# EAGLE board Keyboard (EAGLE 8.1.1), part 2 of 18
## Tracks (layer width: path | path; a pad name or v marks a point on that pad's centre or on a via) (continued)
S$778
  Bottom 0: 246.88,2.82 246.83,2.94
S$779
  Bottom 0: 246.83,2.94 261.31,2.94
S$780
  Bottom 0: 261.31,2.94 261.38,2.95
S$781
  Bottom 0: 261.38,2.95 261.44,2.96
S$782
  Bottom 0: 261.44,2.96 261.51,2.99
S$783
  Bottom 0: 261.51,2.99 261.57,3.03
S$784
  Bottom 0: 261.57,3.03 261.62,3.07
S$785
  Bottom 0: 261.62,3.07 269.2,10.64
S$786
  Bottom 0: 269.2,10.64 269.29,10.6
S$787
  Bottom 0: 269.29,10.6 269.6,10.58
S$788
  Bottom 0: 269.6,10.58 269.89,10.65
S$789
  Bottom 0: 269.89,10.65 270.15,10.8
S$790
  Bottom 0: 270.15,10.8 270.36,11.02
S$791
  Bottom 0: 270.36,11.02 270.44,11.19
S$792
  Bottom 0: 270.44,11.19 270.47,11.14
S$793
  Bottom 0: 270.47,11.14 270.52,11.09
S$794
  Bottom 0: 270.52,11.09 276.91,4.69
S$795
  Bottom 0: 276.91,4.69 276.96,4.65
S$796
  Bottom 0: 276.96,4.65 277.02,4.61
S$797
  Bottom 0: 277.02,4.61 277.09,4.58
S$798
  Bottom 0: 277.09,4.58 277.15,4.56
S$799
  Bottom 0: 277.15,4.56 277.22,4.56
S$800
  Bottom 0: 277.22,4.56 280.74,4.56
S$801
  Bottom 0: 280.74,4.56 280.76,4.49
S$802
  Bottom 0: 280.76,4.49 280.93,4.18
S$803
  Bottom 0: 280.93,4.18 281.17,3.92
S$804
  Bottom 0: 281.17,3.92 281.46,3.74
S$805
  Bottom 0: 281.46,3.74 281.8,3.63
S$806
  Bottom 0: 281.8,3.63 282.15,3.61
S$807
  Bottom 0: 282.15,3.61 282.45,3.67
S$808
  Bottom 0: 282.45,3.67 282.56,3.63
S$809
  Bottom 0: 282.56,3.63 282.91,3.61
S$810
  Bottom 0: 282.91,3.61 283.25,3.67
S$811
  Bottom 0: 283.25,3.67 283.57,3.82
S$812
  Bottom 0: 283.57,3.82 283.84,4.05
S$813
  Bottom 0: 283.84,4.05 284.05,4.33
S$814
  Bottom 0: 284.05,4.33 284.17,4.66
S$815
  Bottom 0: 284.17,4.66 284.22,5
S$816
  Bottom 0: 284.22,5 284.17,5.35
S$817
  Bottom 0: 284.17,5.35 284.05,5.67
S$818
  Bottom 0: 284.05,5.67 283.84,5.96
S$819
  Bottom 0: 283.84,5.96 283.57,6.18
S$820
  Bottom 0: 283.57,6.18 283.25,6.33
S$821
  Bottom 0: 283.25,6.33 282.91,6.39
S$822
  Bottom 0: 282.91,6.39 282.56,6.37
S$823
  Bottom 0: 282.56,6.37 282.45,6.34
S$824
  Bottom 0: 282.45,6.34 282.15,6.39
S$825
  Bottom 0: 282.15,6.39 281.8,6.37
S$826
  Bottom 0: 281.8,6.37 281.46,6.27
S$827
  Bottom 0: 281.46,6.27 281.17,6.08
S$828
  Bottom 0: 281.17,6.08 280.93,5.82
S$829
  Bottom 0: 280.93,5.82 280.76,5.51
S$830
  Bottom 0: 280.76,5.51 280.74,5.44
S$831
  Bottom 0: 280.74,5.44 279.89,5.44
S$832
  Bottom 0: 279.89,5.44 280.27,5.65
S$833
  Bottom 0: 280.27,5.65 280.62,5.93
S$834
  Bottom 0: 280.62,5.93 280.9,6.28
S$835
  Bottom 0: 280.9,6.28 281.12,6.67
S$836
  Bottom 0: 281.12,6.67 281.24,7.1
S$837
  Bottom 0: 281.24,7.1 281.29,7.55
S$838
  Bottom 0: 281.29,7.55 281.24,7.99
S$839
  Bottom 0: 281.24,7.99 281.12,8.42
S$840
  Bottom 0: 281.12,8.42 280.9,8.82
S$841
  Bottom 0: 280.9,8.82 280.62,9.16
S$842
  Bottom 0: 280.62,9.16 280.27,9.45
S$843
  Bottom 0: 280.27,9.45 279.87,9.66
S$844
  Bottom 0: 279.87,9.66 279.62,9.74
S$845
  Bottom 0: 279.62,9.74 284.97,9.74
S$846
  Bottom 0: 284.97,9.74 289.73,4.98
S$847
  Bottom 0: 289.73,4.98 289.53,4.97
S$848
  Bottom 0: 289.53,4.97 289.25,4.85
S$849
  Bottom 0: 289.25,4.85 289.01,4.67
S$850
  Bottom 0: 289.01,4.67 288.85,4.42
S$851
  Bottom 0: 288.85,4.42 288.75,4.13
S$852
  Bottom 0: 288.75,4.13 288.75,3.82
S$853
  Bottom 0: 288.75,3.82 288.85,3.53
S$854
  Bottom 0: 288.85,3.53 289.01,3.28
S$855
  Bottom 0: 289.01,3.28 289.25,3.1
S$856
  Bottom 0: 289.25,3.1 289.53,2.98
S$857
  Bottom 0: 289.53,2.98 289.83,2.96
S$858
  Bottom 0: 289.83,2.96 290.13,3.03
S$859
  Bottom 0: 290.13,3.03 290.4,3.18
S$860
  Bottom 0: 290.4,3.18 290.6,3.4
S$861
  Bottom 0: 290.6,3.4 290.66,3.53
S$862
  Bottom 0: 290.66,3.53 293.86,3.53
S$863
  Bottom 0: 293.86,3.53 293.63,3.28
S$864
  Bottom 0: 293.63,3.28 293.45,2.97
S$865
  Bottom 0: 293.45,2.97 293.43,2.9
S$866
  Bottom 0: 293.43,2.9 289.08,2.9
S$867
  Bottom 0: 289.08,2.9 288.34,3.65
S$868
  Bottom 0: 288.34,3.65 288.35,3.67
S$869
  Bottom 0: 288.35,3.67 288.4,3.98
S$870
  Bottom 0: 288.4,3.98 288.35,4.28
S$871
  Bottom 0: 288.35,4.28 288.22,4.55
S$872
  Bottom 0: 288.22,4.55 288.02,4.77
S$873
  Bottom 0: 288.02,4.77 287.75,4.92
S$874
  Bottom 0: 287.75,4.92 287.46,4.99
S$875
  Bottom 0: 287.46,4.99 287.15,4.97
S$876
  Bottom 0: 287.15,4.97 286.88,4.85
S$877
  Bottom 0: 286.88,4.85 286.64,4.67
S$878
  Bottom 0: 286.64,4.67 286.47,4.42
S$879
  Bottom 0: 286.47,4.42 286.38,4.13
S$880
  Bottom 0: 286.38,4.13 286.38,3.82
S$881
  Bottom 0: 286.38,3.82 286.47,3.53
S$882
  Bottom 0: 286.47,3.53 286.64,3.28
S$883
  Bottom 0: 286.64,3.28 286.88,3.1
S$884
  Bottom 0: 286.88,3.1 287.15,2.98
S$885
  Bottom 0: 287.15,2.98 287.46,2.96
S$886
  Bottom 0: 287.46,2.96 287.71,3.02
S$887
  Bottom 0: 287.71,3.02 288.58,2.15
S$888
  Bottom 0: 288.58,2.15 288.63,2.11
S$889
  Bottom 0: 288.63,2.11 288.7,2.06
S$890
  Bottom 0: 288.7,2.06 288.76,2.04
S$891
  Bottom 0: 288.76,2.04 288.82,2.02
S$892
  Bottom 0: 288.82,2.02 288.9,2.02
S$893
  Bottom 0: 288.9,2.02 293.43,2.02
S$894
  Bottom 0: 293.43,2.02 293.45,1.95
S$895
  Bottom 0: 293.45,1.95 293.63,1.64
S$896
  Bottom 0: 293.63,1.64 293.87,1.38
S$897
  Bottom 0: 293.87,1.38 294.16,1.2
S$898
  Bottom 0: 294.16,1.2 294.49,1.09
S$899
  Bottom 0: 294.49,1.09 294.84,1.07
S$900
  Bottom 0: 294.84,1.07 295.14,1.12
S$901
  Bottom 0: 295.14,1.12 295.25,1.09
S$902
  Bottom 0: 295.25,1.09 295.6,1.07
S$903
  Bottom 0: 295.6,1.07 295.95,1.13
S$904
  Bottom 0: 295.95,1.13 296.26,1.28
S$905
  Bottom 0: 296.26,1.28 296.53,1.51
S$906
  Bottom 0: 296.53,1.51 296.74,1.79
S$907
  Bottom 0: 296.74,1.79 296.87,2.12
S$908
  Bottom 0: 296.87,2.12 296.91,2.46
S$909
  Bottom 0: 296.91,2.46 296.87,2.81
S$910
  Bottom 0: 296.87,2.81 296.74,3.13
S$911
  Bottom 0: 296.74,3.13 296.53,3.42
S$912
  Bottom 0: 296.53,3.42 296.39,3.53
S$913
  Bottom 0: 296.39,3.53 296.52,3.53
S$914
  Bottom 0: 296.52,3.53 296.55,3.49
S$915
  Bottom 0: 296.55,3.49 296.59,3.43
S$916
  Bottom 0: 296.59,3.43 297.44,2.58
S$917
  Bottom 0: 297.44,2.58 297.5,2.54
S$918
  Bottom 0: 297.5,2.54 297.56,2.5
S$919
  Bottom 0: 297.56,2.5 297.62,2.47
S$920
  Bottom 0: 297.62,2.47 297.69,2.46
S$921
  Bottom 0: 297.69,2.46 297.76,2.45
S$922
  Bottom 0: 297.76,2.45 298.36,2.45
S$923
  Bottom 0: 298.36,2.45 298.66,2.15
S$924
  Bottom 0: 298.66,2.15 298.72,2.11
S$925
  Bottom 0: 298.72,2.11 298.78,2.06
S$926
  Bottom 0: 298.78,2.06 298.84,2.04
S$927
  Bottom 0: 298.84,2.04 298.91,2.02
S$928
  Bottom 0: 298.91,2.02 298.98,2.02
S$929
  Bottom 0: 298.98,2.02 312.48,2.02
S$930
  Bottom 0: 312.48,2.02 312.5,1.95
S$931
  Bottom 0: 312.5,1.95 312.67,1.64
S$932
  Bottom 0: 312.67,1.64 312.91,1.38
S$933
  Bottom 0: 312.91,1.38 313.2,1.2
S$934
  Bottom 0: 313.2,1.2 313.54,1.09
S$935
  Bottom 0: 313.54,1.09 313.89,1.07
S$936
  Bottom 0: 313.89,1.07 314.19,1.12
S$937
  Bottom 0: 314.19,1.12 314.3,1.09
S$938
  Bottom 0: 314.3,1.09 314.65,1.07
S$939
  Bottom 0: 314.65,1.07 314.99,1.13
S$940
  Bottom 0: 314.99,1.13 315.31,1.28
S$941
  Bottom 0: 315.31,1.28 315.58,1.51
S$942
  Bottom 0: 315.58,1.51 315.79,1.79
S$943
  Bottom 0: 315.79,1.79 315.91,2.12
S$944
  Bottom 0: 315.91,2.12 315.96,2.46
S$945
  Bottom 0: 315.96,2.46 315.91,2.81
S$946
  Bottom 0: 315.91,2.81 315.79,3.13
S$947
  Bottom 0: 315.79,3.13 315.58,3.42
S$948
  Bottom 0: 315.58,3.42 315.31,3.64
S$949
  Bottom 0: 315.31,3.64 314.99,3.79
S$950
  Bottom 0: 314.99,3.79 314.65,3.85
S$951
  Bottom 0: 314.65,3.85 314.3,3.83
S$952
  Bottom 0: 314.3,3.83 314.19,3.8
S$953
  Bottom 0: 314.19,3.8 313.89,3.85
S$954
  Bottom 0: 313.89,3.85 313.54,3.83
S$955
  Bottom 0: 313.54,3.83 313.2,3.73
S$956
  Bottom 0: 313.2,3.73 312.91,3.54
S$957
  Bottom 0: 312.91,3.54 312.67,3.28
S$958
  Bottom 0: 312.67,3.28 312.5,2.97
S$959
  Bottom 0: 312.5,2.97 312.48,2.9
S$960
  Bottom 0: 312.48,2.9 299.17,2.9
S$961
  Bottom 0: 299.17,2.9 298.86,3.21
S$962
  Bottom 0: 298.86,3.21 298.81,3.25
S$963
  Bottom 0: 298.81,3.25 298.75,3.29
S$964
  Bottom 0: 298.75,3.29 298.69,3.31
S$965
  Bottom 0: 298.69,3.31 298.62,3.33
S$966
  Bottom 0: 298.62,3.33 298.55,3.33
S$967
  Bottom 0: 298.55,3.33 297.94,3.33
S$968
  Bottom 0: 297.94,3.33 297.35,3.93
S$969
  Bottom 0: 297.35,3.93 297.35,3.98
S$970
  Bottom 0: 297.35,3.98 297.32,4.11
S$971
  Bottom 0: 297.32,4.11 297.26,4.23
S$972
  Bottom 0: 297.26,4.23 297.16,4.33
S$973
  Bottom 0: 297.16,4.33 297.04,4.4
S$974
  Bottom 0: 297.04,4.4 296.9,4.42
S$975
  Bottom 0: 296.9,4.42 290.66,4.42
S$976
  Bottom 0: 290.66,4.42 290.6,4.55
S$977
  Bottom 0: 290.6,4.55 290.52,4.63
S$978
  Bottom 0: 290.52,4.63 299.77,4.63
S$979
  Bottom 0: 299.77,4.63 299.8,4.49
S$980
  Bottom 0: 299.8,4.49 299.98,4.18
S$981
  Bottom 0: 299.98,4.18 300.21,3.92
S$982
  Bottom 0: 300.21,3.92 300.51,3.74
S$983
  Bottom 0: 300.51,3.74 300.84,3.63
S$984
  Bottom 0: 300.84,3.63 301.19,3.61
S$985
  Bottom 0: 301.19,3.61 301.5,3.67
S$986
  Bottom 0: 301.5,3.67 301.6,3.63
S$987
  Bottom 0: 301.6,3.63 301.95,3.61
S$988
  Bottom 0: 301.95,3.61 302.3,3.67
S$989
  Bottom 0: 302.3,3.67 302.61,3.82
S$990
  Bottom 0: 302.61,3.82 302.88,4.05
S$991
  Bottom 0: 302.88,4.05 303.09,4.33
S$992
  Bottom 0: 303.09,4.33 303.22,4.66
S$993
  Bottom 0: 303.22,4.66 303.26,5
S$994
  Bottom 0: 303.26,5 303.22,5.35
S$995
  Bottom 0: 303.22,5.35 303.09,5.67
S$996
  Bottom 0: 303.09,5.67 302.88,5.96
S$997
  Bottom 0: 302.88,5.96 302.61,6.18
S$998
  Bottom 0: 302.61,6.18 302.3,6.33
S$999
  Bottom 0: 302.3,6.33 301.95,6.39
S$1000
  Bottom 0: 301.95,6.39 301.6,6.37
S$1001
  Bottom 0: 301.6,6.37 301.5,6.34
S$1002
  Bottom 0: 301.5,6.34 301.19,6.39
S$1003
  Bottom 0: 301.19,6.39 301.02,6.38
S$1004
  Bottom 0: 301.02,6.38 301.02,15.1
S$1005
  Bottom 0: 301.02,15.1 301.22,14.91
S$1006
  Bottom 0: 301.22,14.91 301.51,14.77
S$1007
  Bottom 0: 301.51,14.77 301.83,14.7
S$1008
  Bottom 0: 301.83,14.7 302.15,14.72
S$1009
  Bottom 0: 302.15,14.72 302.46,14.83
S$1010
  Bottom 0: 302.46,14.83 302.73,15.01
S$1011
  Bottom 0: 302.73,15.01 302.93,15.27
S$1012
  Bottom 0: 302.93,15.27 303.06,15.57
S$1013
  Bottom 0: 303.06,15.57 303.11,15.89
S$1014
  Bottom 0: 303.11,15.89 303.06,16.21
S$1015
  Bottom 0: 303.06,16.21 303.05,16.23
S$1016
  Bottom 0: 303.05,16.23 303.75,16.93
S$1017
  Bottom 0: 303.75,16.93 312.77,16.93
S$1018
  Bottom 0: 312.77,16.93 312.65,16.87
S$1019
  Bottom 0: 312.65,16.87 312.42,16.64
S$1020
  Bottom 0: 312.42,16.64 312.25,16.37
S$1021
  Bottom 0: 312.25,16.37 312.16,16.05
S$1022
  Bottom 0: 312.16,16.05 312.16,15.73
S$1023
  Bottom 0: 312.16,15.73 312.25,15.41
S$1024
  Bottom 0: 312.25,15.41 312.42,15.14
S$1025
  Bottom 0: 312.42,15.14 312.65,14.92
S$1026
  Bottom 0: 312.65,14.92 312.94,14.77
S$1027
  Bottom 0: 312.94,14.77 313.26,14.7
S$1028
  Bottom 0: 313.26,14.7 313.58,14.72
S$1029
  Bottom 0: 313.58,14.72 313.61,14.73
S$1030
  Bottom 0: 313.61,14.73 314.57,13.77
S$1031
  Bottom 0: 314.57,13.77 314.19,13.77
S$1032
  Bottom 0: 314.19,13.77 314.11,13.76
S$1033
  Bottom 0: 314.11,13.76 314.04,13.72
S$1034
  Bottom 0: 314.04,13.72 313.98,13.66
S$1035
  Bottom 0: 313.98,13.66 313.94,13.59
S$1036
  Bottom 0: 313.94,13.59 313.93,13.52
S$1037
  Bottom 0: 313.93,13.52 313.93,11.74
S$1038
  Bottom 0: 313.93,11.74 313.94,11.66
S$1039
  Bottom 0: 313.94,11.66 313.98,11.59
S$1040
  Bottom 0: 313.98,11.59 314.04,11.53
S$1041
  Bottom 0: 314.04,11.53 314.11,11.49
S$1042
  Bottom 0: 314.11,11.49 314.19,11.48
S$1043
  Bottom 0: 314.19,11.48 316.59,11.48
S$1044
  Bottom 0: 316.59,11.48 316.67,11.49
S$1045
  Bottom 0: 316.67,11.49 316.74,11.53
S$1046
  Bottom 0: 316.74,11.53 316.8,11.59
S$1047
  Bottom 0: 316.8,11.59 316.84,11.66
S$1048
  Bottom 0: 316.84,11.66 316.85,11.74
S$1049
  Bottom 0: 316.85,11.74 316.85,11.96
S$1050
  Bottom 0: 316.85,11.96 316.86,11.93
S$1051
  Bottom 0: 316.86,11.93 317.1,11.74
S$1052
  Bottom 0: 317.1,11.74 317.38,11.63
S$1053
  Bottom 0: 317.38,11.63 317.69,11.61
S$1054
  Bottom 0: 317.69,11.61 317.81,11.64
S$1055
  Bottom 0: 317.81,11.64 317.9,11.58
S$1056
  Bottom 0: 317.9,11.58 318.21,11.49
S$1057
  Bottom 0: 318.21,11.49 318.53,11.49
S$1058
  Bottom 0: 318.53,11.49 318.84,11.58
S$1059
  Bottom 0: 318.84,11.58 319.12,11.76
S$1060
  Bottom 0: 319.12,11.76 319.33,12
S$1061
  Bottom 0: 319.33,12 319.47,12.3
S$1062
  Bottom 0: 319.47,12.3 319.51,12.62
S$1063
  Bottom 0: 319.51,12.62 319.47,12.94
S$1064
  Bottom 0: 319.47,12.94 319.33,13.24
S$1065
  Bottom 0: 319.33,13.24 319.12,13.48
S$1066
  Bottom 0: 319.12,13.48 318.84,13.66
S$1067
  Bottom 0: 318.84,13.66 318.53,13.75
S$1068
  Bottom 0: 318.53,13.75 318.21,13.75
S$1069
  Bottom 0: 318.21,13.75 317.9,13.66
S$1070
  Bottom 0: 317.9,13.66 317.81,13.61
S$1071
  Bottom 0: 317.81,13.61 317.69,13.63
S$1072
  Bottom 0: 317.69,13.63 317.38,13.61
S$1073
  Bottom 0: 317.38,13.61 317.1,13.5
S$1074
  Bottom 0: 317.1,13.5 316.86,13.31
S$1075
  Bottom 0: 316.86,13.31 316.85,13.29
S$1076
  Bottom 0: 316.85,13.29 316.85,13.52
S$1077
  Bottom 0: 316.85,13.52 316.84,13.59
S$1078
  Bottom 0: 316.84,13.59 316.8,13.66
S$1079
  Bottom 0: 316.8,13.66 316.74,13.72
S$1080
  Bottom 0: 316.74,13.72 316.67,13.76
S$1081
  Bottom 0: 316.67,13.76 316.59,13.77
S$1082
  Bottom 0: 316.59,13.77 315.52,13.77
S$1083
  Bottom 0: 315.52,13.77 315.52,13.89
S$1084
  Bottom 0: 315.52,13.89 315.5,13.95
S$1085
  Bottom 0: 315.5,13.95 315.5,14
S$1086
  Bottom 0: 315.5,14 315.47,14.06
S$1087
  Bottom 0: 315.47,14.06 315.45,14.12
S$1088
  Bottom 0: 315.45,14.12 315.42,14.15
S$1089
  Bottom 0: 315.42,14.15 315.39,14.2
S$1090
  Bottom 0: 315.39,14.2 314.34,15.25
S$1091
  Bottom 0: 314.34,15.25 314.36,15.27
S$1092
  Bottom 0: 314.36,15.27 314.49,15.57
S$1093
  Bottom 0: 314.49,15.57 314.54,15.89
S$1094
  Bottom 0: 314.54,15.89 314.49,16.21
S$1095
  Bottom 0: 314.49,16.21 314.36,16.51
S$1096
  Bottom 0: 314.36,16.51 314.15,16.77
S$1097
  Bottom 0: 314.15,16.77 313.93,16.93
S$1098
  Bottom 0: 313.93,16.93 319.12,16.93
S$1099
  Bottom 0: 319.12,16.93 319.82,16.23
S$1100
  Bottom 0: 319.82,16.23 319.78,16.05
S$1101
  Bottom 0: 319.78,16.05 319.78,15.73
S$1102
  Bottom 0: 319.78,15.73 319.87,15.41
S$1103
  Bottom 0: 319.87,15.41 320.04,15.14
S$1104
  Bottom 0: 320.04,15.14 320.27,14.92
S$1105
  Bottom 0: 320.27,14.92 320.56,14.77
S$1106
  Bottom 0: 320.56,14.77 320.88,14.7
S$1107
  Bottom 0: 320.88,14.7 321.2,14.72
S$1108
  Bottom 0: 321.2,14.72 321.51,14.83
S$1109
  Bottom 0: 321.51,14.83 321.77,15.02
S$1110
  Bottom 0: 321.77,15.02 321.84,15.1
S$1111
  Bottom 0: 321.84,15.1 321.84,7.32
S$1112
  Bottom 0: 321.84,7.32 320.91,6.39
S$1113
  Bottom 0: 320.91,6.39 320.65,6.37
S$1114
  Bottom 0: 320.65,6.37 320.54,6.34
S$1115
  Bottom 0: 320.54,6.34 320.24,6.39
S$1116
  Bottom 0: 320.24,6.39 319.88,6.37
S$1117
  Bottom 0: 319.88,6.37 319.55,6.27
S$1118
  Bottom 0: 319.55,6.27 319.26,6.08
S$1119
  Bottom 0: 319.26,6.08 319.02,5.82
S$1120
  Bottom 0: 319.02,5.82 318.85,5.51
S$1121
  Bottom 0: 318.85,5.51 318.76,5.17
S$1122
  Bottom 0: 318.76,5.17 318.76,4.83
S$1123
  Bottom 0: 318.76,4.83 318.85,4.49
S$1124
  Bottom 0: 318.85,4.49 319.02,4.18
S$1125
  Bottom 0: 319.02,4.18 319.26,3.92
S$1126
  Bottom 0: 319.26,3.92 319.55,3.74
S$1127
  Bottom 0: 319.55,3.74 319.88,3.63
S$1128
  Bottom 0: 319.88,3.63 320.24,3.61
S$1129
  Bottom 0: 320.24,3.61 320.54,3.67
S$1130
  Bottom 0: 320.54,3.67 320.65,3.63
S$1131
  Bottom 0: 320.65,3.63 321,3.61
S$1132
  Bottom 0: 321,3.61 321.34,3.67
S$1133
  Bottom 0: 321.34,3.67 321.65,3.82
S$1134
  Bottom 0: 321.65,3.82 321.93,4.05
S$1135
  Bottom 0: 321.93,4.05 322.13,4.33
S$1136
  Bottom 0: 322.13,4.33 322.26,4.66
S$1137
  Bottom 0: 322.26,4.66 322.31,5
S$1138
  Bottom 0: 322.31,5 322.26,5.35
S$1139
  Bottom 0: 322.26,5.35 322.13,5.67
S$1140
  Bottom 0: 322.13,5.67 321.93,5.96
S$1141
  Bottom 0: 321.93,5.96 321.81,6.05
S$1142
  Bottom 0: 321.81,6.05 322.59,6.83
S$1143
  Bottom 0: 322.59,6.83 322.63,6.88
S$1144
  Bottom 0: 322.63,6.88 322.67,6.94
S$1145
  Bottom 0: 322.67,6.94 322.7,7
S$1146
  Bottom 0: 322.7,7 322.71,7.06
S$1147
  Bottom 0: 322.71,7.06 322.72,7.13
S$1148
  Bottom 0: 322.72,7.13 322.72,26.22
S$1149
  Bottom 0: 322.72,26.22 323.52,26.22
S$1150
  Bottom 0: 323.52,26.22 323.6,26.23
S$1151
  Bottom 0: 323.6,26.23 323.67,26.27
S$1152
  Bottom 0: 323.67,26.27 323.73,26.33
S$1153
  Bottom 0: 323.73,26.33 323.77,26.4
S$1154
  Bottom 0: 323.77,26.4 323.78,26.47
S$1155
  Bottom 0: 323.78,26.47 323.78,54.3
S$1156
  Bottom 0: 323.78,54.3 323.77,54.37
S$1157
  Bottom 0: 323.77,54.37 323.73,54.45
S$1158
  Bottom 0: 323.73,54.45 323.67,54.5
S$1159
  Bottom 0: 323.67,54.5 323.6,54.54
S$1160
  Bottom 0: 323.6,54.54 323.52,54.55
S$1161
  Bottom 0: 323.52,54.55 322.72,54.55
S$1162
  Bottom 0: 322.72,54.55 322.72,60.78
S$1163
  Bottom 0: 322.72,60.78 322.71,60.86
S$1164
  Bottom 0: 322.71,60.86 322.7,60.92
S$1165
  Bottom 0: 322.7,60.92 322.67,60.98
S$1166
  Bottom 0: 322.67,60.98 322.63,61.04
S$1167
  Bottom 0: 322.63,61.04 322.59,61.09
S$1168
  Bottom 0: 322.59,61.09 322.16,61.53
S$1169
  Bottom 0: 322.16,61.53 322.27,61.81
S$1170
  Bottom 0: 322.27,61.81 322.31,62.15
S$1171
  Bottom 0: 322.31,62.15 322.27,62.49
S$1172
  Bottom 0: 322.27,62.49 322.14,62.82
S$1173
  Bottom 0: 322.14,62.82 321.93,63.11
S$1174
  Bottom 0: 321.93,63.11 321.66,63.33
S$1175
  Bottom 0: 321.66,63.33 321.35,63.48
S$1176
  Bottom 0: 321.35,63.48 321,63.54
S$1177
  Bottom 0: 321,63.54 320.65,63.52
S$1178
  Bottom 0: 320.65,63.52 320.55,63.49
S$1179
  Bottom 0: 320.55,63.49 320.24,63.54
S$1180
  Bottom 0: 320.24,63.54 320,63.53
S$1181
  Bottom 0: 320,63.53 322.81,66.34
S$1182
  Bottom 0: 322.81,66.34 322.85,66.39
S$1183
  Bottom 0: 322.85,66.39 322.89,66.45
S$1184
  Bottom 0: 322.89,66.45 322.91,66.52
S$1185
  Bottom 0: 322.91,66.52 322.93,66.58
S$1186
  Bottom 0: 322.93,66.58 322.93,66.65
S$1187
  Bottom 0: 322.93,66.65 322.93,81.77
S$1188
  Bottom 0: 322.93,81.77 322.93,81.84
S$1189
  Bottom 0: 322.93,81.84 322.91,81.91
S$1190
  Bottom 0: 322.91,81.91 322.89,81.97
S$1191
  Bottom 0: 322.89,81.97 322.85,82.03
S$1192
  Bottom 0: 322.85,82.03 322.81,82.08
S$1193
  Bottom 0: 322.81,82.08 318.37,86.53
S$1194
  Bottom 0: 318.37,86.53 318.38,86.57
S$1195
  Bottom 0: 318.38,86.57 318.33,86.82
S$1196
  Bottom 0: 318.33,86.82 318.2,87.03
S$1197
  Bottom 0: 318.2,87.03 318,87.19
S$1198
  Bottom 0: 318,87.19 317.75,87.25
S$1199
  Bottom 0: 317.75,87.25 317.5,87.23
S$1200
  Bottom 0: 317.5,87.23 317.38,87.17
S$1201
  Bottom 0: 317.38,87.17 317.97,87.76
S$1202
  Bottom 0: 317.97,87.76 318.21,87.69
S$1203
  Bottom 0: 318.21,87.69 318.54,87.69
S$1204
  Bottom 0: 318.54,87.69 318.85,87.78
S$1205
  Bottom 0: 318.85,87.78 319.12,87.96
S$1206
  Bottom 0: 319.12,87.96 319.34,88.2
S$1207
  Bottom 0: 319.34,88.2 319.47,88.5
S$1208
  Bottom 0: 319.47,88.5 319.52,88.82
S$1209
  Bottom 0: 319.52,88.82 319.47,89.14
S$1210
  Bottom 0: 319.47,89.14 319.34,89.44
S$1211
  Bottom 0: 319.34,89.44 319.12,89.69
S$1212
  Bottom 0: 319.12,89.69 318.85,89.86
S$1213
  Bottom 0: 318.85,89.86 318.54,89.95
S$1214
  Bottom 0: 318.54,89.95 318.21,89.95
S$1215
  Bottom 0: 318.21,89.95 318,89.89
S$1216
  Bottom 0: 318,89.89 317.27,90.61
S$1217
  Bottom 0: 317.27,90.61 317.2,90.67
S$1218
  Bottom 0: 317.2,90.67 317.13,90.72
S$1219
  Bottom 0: 317.13,90.72 317.05,90.75
S$1220
  Bottom 0: 317.05,90.75 316.96,90.77
S$1221
  Bottom 0: 316.96,90.77 316.87,90.78
S$1222
  Bottom 0: 316.87,90.78 300.71,90.78
S$1223
  Bottom 0: 300.71,90.78 300.62,90.77
S$1224
  Bottom 0: 300.62,90.77 300.53,90.75
S$1225
  Bottom 0: 300.53,90.75 300.45,90.72
S$1226
  Bottom 0: 300.45,90.72 300.37,90.67
S$1227
  Bottom 0: 300.37,90.67 300.31,90.61
S$1228
  Bottom 0: 300.31,90.61 299.61,89.91
S$1229
  Bottom 0: 299.61,89.91 299.48,89.95
S$1230
  Bottom 0: 299.48,89.95 299.16,89.95
S$1231
  Bottom 0: 299.16,89.95 298.94,89.89
S$1232
  Bottom 0: 298.94,89.89 298.22,90.61
S$1233
  Bottom 0: 298.22,90.61 298.15,90.67
S$1234
  Bottom 0: 298.15,90.67 298.08,90.72
S$1235
  Bottom 0: 298.08,90.72 298,90.75
S$1236
  Bottom 0: 298,90.75 297.91,90.77
S$1237
  Bottom 0: 297.91,90.77 297.82,90.78
S$1238
  Bottom 0: 297.82,90.78 289.15,90.78
S$1239
  Bottom 0: 289.15,90.78 289.06,90.77
S$1240
  Bottom 0: 289.06,90.77 288.97,90.75
S$1241
  Bottom 0: 288.97,90.75 288.89,90.72
S$1242
  Bottom 0: 288.89,90.72 288.82,90.67
S$1243
  Bottom 0: 288.82,90.67 288.75,90.61
S$1244
  Bottom 0: 288.75,90.61 283.83,85.69
S$1245
  Bottom 0: 283.83,85.69 283.77,85.62
S$1246
  Bottom 0: 283.77,85.62 283.72,85.55
S$1247
  Bottom 0: 283.72,85.55 283.68,85.46
S$1248
  Bottom 0: 283.68,85.46 283.67,85.38
S$1249
  Bottom 0: 283.67,85.38 283.66,85.29
S$1250
  Bottom 0: 283.66,85.29 283.66,83.92
S$1251
  Bottom 0: 283.66,83.92 283.6,83.88
S$1252
  Bottom 0: 283.6,83.88 283.54,83.82
S$1253
  Bottom 0: 283.54,83.82 281.79,82.08
S$1254
  Bottom 0: 281.79,82.08 281.73,82.01
S$1255
  Bottom 0: 281.73,82.01 281.68,81.93
S$1256
  Bottom 0: 281.68,81.93 281.64,81.85
S$1257
  Bottom 0: 281.64,81.85 281.63,81.77
S$1258
  Bottom 0: 281.63,81.77 281.62,81.67
S$1259
  Bottom 0: 281.62,81.67 281.62,77.38
S$1260
  Bottom 0: 281.62,77.38 276.76,77.38
S$1261
  Bottom 0: 276.76,77.38 276.76,79.22
S$1262
  Bottom 0: 276.76,79.22 276.75,79.31
S$1263
  Bottom 0: 276.75,79.31 276.74,79.39
S$1264
  Bottom 0: 276.74,79.39 276.7,79.47
S$1265
  Bottom 0: 276.7,79.47 276.65,79.55
S$1266
  Bottom 0: 276.65,79.55 276.59,79.62
S$1267
  Bottom 0: 276.59,79.62 267.11,89.1
S$1268
  Bottom 0: 267.11,89.1 267.1,89.16
S$1269
  Bottom 0: 267.1,89.16 266.96,89.46
S$1270
  Bottom 0: 266.96,89.46 266.75,89.7
S$1271
  Bottom 0: 266.75,89.7 266.47,89.88
S$1272
  Bottom 0: 266.47,89.88 266.16,89.97
S$1273
  Bottom 0: 266.16,89.97 265.84,89.97
S$1274
  Bottom 0: 265.84,89.97 265.53,89.88
S$1275
  Bottom 0: 265.53,89.88 265.25,89.7
S$1276
  Bottom 0: 265.25,89.7 265.04,89.46
S$1277
  Bottom 0: 265.04,89.46 264.9,89.16
S$1278
  Bottom 0: 264.9,89.16 264.86,88.84
S$1279
  Bottom 0: 264.86,88.84 264.9,88.54
S$1280
  Bottom 0: 264.9,88.54 264.6,88.24
S$1281
  Bottom 0: 264.6,88.24 264.6,89.72
S$1282
  Bottom 0: 264.6,89.72 264.59,89.8
S$1283
  Bottom 0: 264.59,89.8 264.55,89.87
S$1284
  Bottom 0: 264.55,89.87 264.5,89.93
S$1285
  Bottom 0: 264.5,89.93 264.43,89.97
S$1286
  Bottom 0: 264.43,89.97 264.35,89.98
S$1287
  Bottom 0: 264.35,89.98 262.57,89.98
S$1288
  Bottom 0: 262.57,89.98 262.5,89.97
S$1289
  Bottom 0: 262.5,89.97 262.43,89.93
S$1290
  Bottom 0: 262.43,89.93 262.37,89.87
S$1291
  Bottom 0: 262.37,89.87 262.33,89.8
S$1292
  Bottom 0: 262.33,89.8 262.32,89.72
S$1293
  Bottom 0: 262.32,89.72 262.32,88.02
S$1294
  Bottom 0: 262.32,88.02 247.74,88.02
S$1295
  Bottom 0: 247.74,88.02 246.22,89.53
S$1296
  Bottom 0: 246.22,89.53 246.16,89.59
S$1297
  Bottom 0: 246.16,89.59 246.08,89.64
S$1298
  Bottom 0: 246.08,89.64 246,89.67
S$1299
  Bottom 0: 246,89.67 245.91,89.69
S$1300
  Bottom 0: 245.91,89.69 245.82,89.7
S$1301
  Bottom 0: 245.82,89.7 238.17,89.7
S$1302
  Bottom 0: 238.17,89.7 237.9,89.88
S$1303
  Bottom 0: 237.9,89.88 237.59,89.97
S$1304
  Bottom 0: 237.59,89.97 237.26,89.97
S$1305
  Bottom 0: 237.26,89.97 236.95,89.88
S$1306
  Bottom 0: 236.95,89.88 236.68,89.7
S$1307
  Bottom 0: 236.68,89.7 236.47,89.46
S$1308
  Bottom 0: 236.47,89.46 236.33,89.16
S$1309
  Bottom 0: 236.33,89.16 236.28,88.84
S$1310
  Bottom 0: 236.28,88.84 236.33,88.52
S$1311
  Bottom 0: 236.33,88.52 236.47,88.22
S$1312
  Bottom 0: 236.47,88.22 236.68,87.97
S$1313
  Bottom 0: 236.68,87.97 236.95,87.8
S$1314
  Bottom 0: 236.95,87.8 237.26,87.7
S$1315
  Bottom 0: 237.26,87.7 237.59,87.7
S$1316
  Bottom 0: 237.59,87.7 237.9,87.8
S$1317
  Bottom 0: 237.9,87.8 238.17,87.97
S$1318
  Bottom 0: 238.17,87.97 238.39,88.22
S$1319
  Bottom 0: 238.39,88.22 238.52,88.52
S$1320
  Bottom 0: 238.52,88.52 238.53,88.56
S$1321
  Bottom 0: 238.53,88.56 243.86,88.56
S$1322
  Bottom 0: 243.86,88.56 243.77,88.5
S$1323
  Bottom 0: 243.77,88.5 243.6,88.25
S$1324
  Bottom 0: 243.6,88.25 243.51,87.96
S$1325
  Bottom 0: 243.51,87.96 243.51,87.65
S$1326
  Bottom 0: 243.51,87.65 243.52,87.63
S$1327
  Bottom 0: 243.52,87.63 238.08,82.18
S$1328
  Bottom 0: 238.08,82.18 238.04,82.13
S$1329
  Bottom 0: 238.04,82.13 238,82.06
S$1330
  Bottom 0: 238,82.06 237.97,82
S$1331
  Bottom 0: 237.97,82 237.96,81.94
S$1332
  Bottom 0: 237.96,81.94 237.95,81.87
S$1333
  Bottom 0: 237.95,81.87 237.95,79.34
S$1334
  Bottom 0: 237.95,79.34 237.96,79.27
S$1335
  Bottom 0: 237.96,79.27 237.97,79.2
S$1336
  Bottom 0: 237.97,79.2 238,79.14
S$1337
  Bottom 0: 238,79.14 238.04,79.08
S$1338
  Bottom 0: 238.04,79.08 238.08,79.03
S$1339
  Bottom 0: 238.08,79.03 245.24,71.86
S$1340
  Bottom 0: 245.24,71.86 245.24,70.93
S$1341
  Bottom 0: 245.24,70.93 244.85,70.93
S$1342
  Bottom 0: 244.85,70.93 244.85,71.06
S$1343
  Bottom 0: 244.85,71.06 244.79,71.28
S$1344
  Bottom 0: 244.79,71.28 244.63,71.44
S$1345
  Bottom 0: 244.63,71.44 244.41,71.5
S$1346
  Bottom 0: 244.41,71.5 244.07,71.5
S$1347
  Bottom 0: 244.07,71.5 242.98,72.59
S$1348
  Bottom 0: 242.98,72.59 243.04,72.72
S$1349
  Bottom 0: 243.04,72.72 243.09,73.04
S$1350
  Bottom 0: 243.09,73.04 243.04,73.36
S$1351
  Bottom 0: 243.04,73.36 242.91,73.66
S$1352
  Bottom 0: 242.91,73.66 242.71,73.92
S$1353
  Bottom 0: 242.71,73.92 242.45,74.11
S$1354
  Bottom 0: 242.45,74.11 242.14,74.21
S$1355
  Bottom 0: 242.14,74.21 241.82,74.23
S$1356
  Bottom 0: 241.82,74.23 241.5,74.17
S$1357
  Bottom 0: 241.5,74.17 241.21,74.02
S$1358
  Bottom 0: 241.21,74.02 240.97,73.8
S$1359
  Bottom 0: 240.97,73.8 240.8,73.52
S$1360
  Bottom 0: 240.8,73.52 240.71,73.2
S$1361
  Bottom 0: 240.71,73.2 240.71,72.88
S$1362
  Bottom 0: 240.71,72.88 240.8,72.56
S$1363
  Bottom 0: 240.8,72.56 240.97,72.29
S$1364
  Bottom 0: 240.97,72.29 241.21,72.07
S$1365
  Bottom 0: 241.21,72.07 241.5,71.92
S$1366
  Bottom 0: 241.5,71.92 241.82,71.85
S$1367
  Bottom 0: 241.82,71.85 242.14,71.87
S$1368
  Bottom 0: 242.14,71.87 242.36,71.95
S$1369
  Bottom 0: 242.36,71.95 243.41,70.9
S$1370
  Bottom 0: 243.41,70.9 243.38,70.88
S$1371
  Bottom 0: 243.38,70.88 243.32,70.82
S$1372
  Bottom 0: 243.32,70.82 243.28,70.75
S$1373
  Bottom 0: 243.28,70.75 243.27,70.67
S$1374
  Bottom 0: 243.27,70.67 243.27,68.9
S$1375
  Bottom 0: 243.27,68.9 243.28,68.82
S$1376
  Bottom 0: 243.28,68.82 243.32,68.75
S$1377
  Bottom 0: 243.32,68.75 243.38,68.69
S$1378
  Bottom 0: 243.38,68.69 243.45,68.65
S$1379
  Bottom 0: 243.45,68.65 243.52,68.64
S$1380
  Bottom 0: 243.52,68.64 245.3,68.64
S$1381
  Bottom 0: 245.3,68.64 245.38,68.65
S$1382
  Bottom 0: 245.38,68.65 245.45,68.69
S$1383
  Bottom 0: 245.45,68.69 245.47,68.72
S$1384
  Bottom 0: 245.47,68.72 245.99,68.2
S$1385
  Bottom 0: 245.99,68.2 237.79,68.2
S$1386
  Bottom 0: 237.79,68.2 226.8,79.19
S$1387
  Bottom 0: 226.8,79.19 227.02,79.24
S$1388
  Bottom 0: 227.02,79.24 227.29,79.39
S$1389
  Bottom 0: 227.29,79.39 227.49,79.61
S$1390
  Bottom 0: 227.49,79.61 227.62,79.89
S$1391
  Bottom 0: 227.62,79.89 227.67,80.19
S$1392
  Bottom 0: 227.67,80.19 227.62,80.48
S$1393
  Bottom 0: 227.62,80.48 227.49,80.76
S$1394
  Bottom 0: 227.49,80.76 227.29,80.98
S$1395
  Bottom 0: 227.29,80.98 227.09,81.09
S$1396
  Bottom 0: 227.09,81.09 227.09,82.51
S$1397
  Bottom 0: 227.09,82.51 227.09,82.58
S$1398
  Bottom 0: 227.09,82.58 227.07,82.65
S$1399
  Bottom 0: 227.07,82.65 227.05,82.71
S$1400
  Bottom 0: 227.05,82.71 227.01,82.77
S$1401
  Bottom 0: 227.01,82.77 226.97,82.83
S$1402
  Bottom 0: 226.97,82.83 219.25,90.54
S$1403
  Bottom 0: 219.25,90.54 219.2,90.58
S$1404
  Bottom 0: 219.2,90.58 219.14,90.62
S$1405
  Bottom 0: 219.14,90.62 219.08,90.64
S$1406
  Bottom 0: 219.08,90.64 219.01,90.66
S$1407
  Bottom 0: 219.01,90.66 218.94,90.67
S$1408
  Bottom 0: 218.94,90.67 217.98,90.67
S$1409
  Bottom 0: 217.98,90.67 217.91,90.66
S$1410
  Bottom 0: 217.91,90.66 217.84,90.64
S$1411
  Bottom 0: 217.84,90.64 217.78,90.62
S$1412
  Bottom 0: 217.78,90.62 217.72,90.58
S$1413
  Bottom 0: 217.72,90.58 217.66,90.54
S$1414
  Bottom 0: 217.66,90.54 216.95,89.83
S$1415
  Bottom 0: 216.95,89.83 216.93,89.87
S$1416
  Bottom 0: 216.93,89.87 216.87,89.93
S$1417
  Bottom 0: 216.87,89.93 216.8,89.97
S$1418
  Bottom 0: 216.8,89.97 216.73,89.98
S$1419
  Bottom 0: 216.73,89.98 214.95,89.98
S$1420
  Bottom 0: 214.95,89.98 214.87,89.97
S$1421
  Bottom 0: 214.87,89.97 214.8,89.93
S$1422
  Bottom 0: 214.8,89.93 214.74,89.87
S$1423
  Bottom 0: 214.74,89.87 214.7,89.8
S$1424
  Bottom 0: 214.7,89.8 214.69,89.72
S$1425
  Bottom 0: 214.69,89.72 214.69,87.95
S$1426
  Bottom 0: 214.69,87.95 214.7,87.87
S$1427
  Bottom 0: 214.7,87.87 214.74,87.8
S$1428
  Bottom 0: 214.74,87.8 214.8,87.74
S$1429
  Bottom 0: 214.8,87.74 214.87,87.7
S$1430
  Bottom 0: 214.87,87.7 214.95,87.69
S$1431
  Bottom 0: 214.95,87.69 215.33,87.69
S$1432
  Bottom 0: 215.33,87.69 212.68,85.05
S$1433
  Bottom 0: 212.68,85.05 212.65,84.99
S$1434
  Bottom 0: 212.65,84.99 212.61,84.93
S$1435
  Bottom 0: 212.61,84.93 212.58,84.87
S$1436
  Bottom 0: 212.58,84.87 212.56,84.8
S$1437
  Bottom 0: 212.56,84.8 212.56,84.73
S$1438
  Bottom 0: 212.56,84.73 212.56,76.33
S$1439
  Bottom 0: 212.56,76.33 212.39,76.17
S$1440
  Bottom 0: 212.39,76.17 212.22,75.89
S$1441
  Bottom 0: 212.22,75.89 212.13,75.58
S$1442
  Bottom 0: 212.13,75.58 212.13,75.25
S$1443
  Bottom 0: 212.13,75.25 212.22,74.94
S$1444
  Bottom 0: 212.22,74.94 212.3,74.81
S$1445
  Bottom 0: 212.3,74.81 209.58,77.52
S$1446
  Bottom 0: 209.58,77.52 209.53,77.56
S$1447
  Bottom 0: 209.53,77.56 209.47,77.61
S$1448
  Bottom 0: 209.47,77.61 209.41,77.63
S$1449
  Bottom 0: 209.41,77.63 209.34,77.64
S$1450
  Bottom 0: 209.34,77.64 209.27,77.65
S$1451
  Bottom 0: 209.27,77.65 206.05,77.65
S$1452
  Bottom 0: 206.05,77.65 203.11,80.6
S$1453
  Bottom 0: 203.11,80.6 203.22,80.87
S$1454
  Bottom 0: 203.22,80.87 203.26,81.22
S$1455
  Bottom 0: 203.26,81.22 203.22,81.56
S$1456
  Bottom 0: 203.22,81.56 203.09,81.89
S$1457
  Bottom 0: 203.09,81.89 202.88,82.17
S$1458
  Bottom 0: 202.88,82.17 202.61,82.39
S$1459
  Bottom 0: 202.61,82.39 202.3,82.55
S$1460
  Bottom 0: 202.3,82.55 201.95,82.61
S$1461
  Bottom 0: 201.95,82.61 201.6,82.59
S$1462
  Bottom 0: 201.6,82.59 201.27,82.48
S$1463
  Bottom 0: 201.27,82.48 200.98,82.29
S$1464
  Bottom 0: 200.98,82.29 200.74,82.04
S$1465
  Bottom 0: 200.74,82.04 200.74,82.06
S$1466
  Bottom 0: 200.74,82.06 200.98,82.31
S$1467
  Bottom 0: 200.98,82.31 201.04,82.38
S$1468
  Bottom 0: 201.04,82.38 201.09,82.45
S$1469
  Bottom 0: 201.09,82.45 201.12,82.53
S$1470
  Bottom 0: 201.12,82.53 201.15,82.62
S$1471
  Bottom 0: 201.15,82.62 201.15,82.71
S$1472
  Bottom 0: 201.15,82.71 201.15,87.58
S$1473
  Bottom 0: 201.15,87.58 201.15,87.66
S$1474
  Bottom 0: 201.15,87.66 201.12,87.75
S$1475
  Bottom 0: 201.12,87.75 201.09,87.84
S$1476
  Bottom 0: 201.09,87.84 201.04,87.91
S$1477
  Bottom 0: 201.04,87.91 200.98,87.98
S$1478
  Bottom 0: 200.98,87.98 200.43,88.54
S$1479
  Bottom 0: 200.43,88.54 200.47,88.84
S$1480
  Bottom 0: 200.47,88.84 200.42,89.16
S$1481
  Bottom 0: 200.42,89.16 200.29,89.46
S$1482
  Bottom 0: 200.29,89.46 200.07,89.7
S$1483
  Bottom 0: 200.07,89.7 199.8,89.88
S$1484
  Bottom 0: 199.8,89.88 199.49,89.97
S$1485
  Bottom 0: 199.49,89.97 199.16,89.97
S$1486
  Bottom 0: 199.16,89.97 198.85,89.88
S$1487
  Bottom 0: 198.85,89.88 198.58,89.7
S$1488
  Bottom 0: 198.58,89.7 198.48,89.59
S$1489
  Bottom 0: 198.48,89.59 198.48,89.98
S$1490
  Bottom 0: 198.48,89.98 198.48,90.06
S$1491
  Bottom 0: 198.48,90.06 198.46,90.12
S$1492
  Bottom 0: 198.46,90.12 198.44,90.18
S$1493
  Bottom 0: 198.44,90.18 198.39,90.24
S$1494
  Bottom 0: 198.39,90.24 198.36,90.3
S$1495
  Bottom 0: 198.36,90.3 198.24,90.41
S$1496
  Bottom 0: 198.24,90.41 198.19,90.45
S$1497
  Bottom 0: 198.19,90.45 198.13,90.49
S$1498
  Bottom 0: 198.13,90.49 198.07,90.52
S$1499
  Bottom 0: 198.07,90.52 198,90.53
S$1500
  Bottom 0: 198,90.53 197.93,90.54
S$1501
  Bottom 0: 197.93,90.54 195.67,90.54
S$1502
  Bottom 0: 195.67,90.54 195.6,90.53
S$1503
  Bottom 0: 195.6,90.53 195.53,90.52
S$1504
  Bottom 0: 195.53,90.52 195.47,90.49
S$1505
  Bottom 0: 195.47,90.49 195.35,90.41
S$1506
  Bottom 0: 195.35,90.41 186.61,81.66
S$1507
  Bottom 0: 186.61,81.66 184.13,81.66
S$1508
  Bottom 0: 184.13,81.66 184.04,81.89
S$1509
  Bottom 0: 184.04,81.89 183.83,82.17
S$1510
  Bottom 0: 183.83,82.17 183.56,82.39
S$1511
  Bottom 0: 183.56,82.39 183.25,82.55
S$1512
  Bottom 0: 183.25,82.55 182.9,82.61
S$1513
  Bottom 0: 182.9,82.61 182.55,82.59
S$1514
  Bottom 0: 182.55,82.59 182.22,82.48
S$1515
  Bottom 0: 182.22,82.48 181.93,82.29
S$1516
  Bottom 0: 181.93,82.29 181.69,82.04
S$1517
  Bottom 0: 181.69,82.04 181.52,81.73
S$1518
  Bottom 0: 181.52,81.73 181.43,81.39
S$1519
  Bottom 0: 181.43,81.39 181.43,81.04
S$1520
  Bottom 0: 181.43,81.04 181.52,80.7
S$1521
  Bottom 0: 181.52,80.7 181.69,80.39
S$1522
  Bottom 0: 181.69,80.39 181.93,80.14
S$1523
  Bottom 0: 181.93,80.14 182.22,79.95
S$1524
  Bottom 0: 182.22,79.95 182.55,79.84
S$1525
  Bottom 0: 182.55,79.84 182.9,79.83
S$1526
  Bottom 0: 182.9,79.83 183.25,79.89
S$1527
  Bottom 0: 183.25,79.89 183.56,80.04
S$1528
  Bottom 0: 183.56,80.04 183.83,80.26
S$1529
  Bottom 0: 183.83,80.26 184.04,80.55
S$1530
  Bottom 0: 184.04,80.55 184.13,80.78
S$1531
  Bottom 0: 184.13,80.78 186.55,80.78
S$1532
  Bottom 0: 186.55,80.78 186.45,80.63
S$1533
  Bottom 0: 186.45,80.63 186.36,80.34
S$1534
  Bottom 0: 186.36,80.34 186.36,80.03
S$1535
  Bottom 0: 186.36,80.03 186.45,79.74
S$1536
  Bottom 0: 186.45,79.74 186.62,79.49
S$1537
  Bottom 0: 186.62,79.49 186.85,79.31
S$1538
  Bottom 0: 186.85,79.31 187.13,79.19
S$1539
  Bottom 0: 187.13,79.19 187.44,79.17
S$1540
  Bottom 0: 187.44,79.17 187.73,79.24
S$1541
  Bottom 0: 187.73,79.24 188,79.39
S$1542
  Bottom 0: 188,79.39 188.2,79.61
S$1543
  Bottom 0: 188.2,79.61 188.33,79.89
S$1544
  Bottom 0: 188.33,79.89 188.38,80.19
S$1545
  Bottom 0: 188.38,80.19 188.33,80.48
S$1546
  Bottom 0: 188.33,80.48 188.2,80.76
S$1547
  Bottom 0: 188.2,80.76 188,80.98
S$1548
  Bottom 0: 188,80.98 187.73,81.13
S$1549
  Bottom 0: 187.73,81.13 187.44,81.2
S$1550
  Bottom 0: 187.44,81.2 187.4,81.19
S$1551
  Bottom 0: 187.4,81.19 195.64,89.44
S$1552
  Bottom 0: 195.64,89.44 195.64,87.95
S$1553
  Bottom 0: 195.64,87.95 195.65,87.87
S$1554
  Bottom 0: 195.65,87.87 195.69,87.8
S$1555
  Bottom 0: 195.69,87.8 195.75,87.74
S$1556
  Bottom 0: 195.75,87.74 195.82,87.7
S$1557
  Bottom 0: 195.82,87.7 195.9,87.69
S$1558
  Bottom 0: 195.9,87.69 196.29,87.69
S$1559
  Bottom 0: 196.29,87.69 193.56,84.97
S$1560
  Bottom 0: 193.56,84.97 193.51,84.92
S$1561
  Bottom 0: 193.51,84.92 193.48,84.86
S$1562
  Bottom 0: 193.48,84.86 193.45,84.79
S$1563
  Bottom 0: 193.45,84.79 193.43,84.73
S$1564
  Bottom 0: 193.43,84.73 193.43,84.66
S$1565
  Bottom 0: 193.43,84.66 193.43,76.25
S$1566
  Bottom 0: 193.43,76.25 193.34,76.17
S$1567
  Bottom 0: 193.34,76.17 193.17,75.89
S$1568
  Bottom 0: 193.17,75.89 193.08,75.58
S$1569
  Bottom 0: 193.08,75.58 193.08,75.25
S$1570
  Bottom 0: 193.08,75.25 193.17,74.94
S$1571
  Bottom 0: 193.17,74.94 193.25,74.81
S$1572
  Bottom 0: 193.25,74.81 190.98,77.08
S$1573
  Bottom 0: 190.98,77.08 190.93,77.12
S$1574
  Bottom 0: 190.93,77.12 190.87,77.16
S$1575
  Bottom 0: 190.87,77.16 190.81,77.18
S$1576
  Bottom 0: 190.81,77.18 190.74,77.2
S$1577
  Bottom 0: 190.74,77.2 190.67,77.2
S$1578
  Bottom 0: 190.67,77.2 181.09,77.2
S$1579
  Bottom 0: 181.09,77.2 181.02,77.2
S$1580
  Bottom 0: 181.02,77.2 180.95,77.18
S$1581
  Bottom 0: 180.95,77.18 180.89,77.16
S$1582
  Bottom 0: 180.89,77.16 180.83,77.12
S$1583
  Bottom 0: 180.83,77.12 180.77,77.08
S$1584
  Bottom 0: 180.77,77.08 178.24,74.55
S$1585
  Bottom 0: 178.24,74.55 176.03,74.55
S$1586
  Bottom 0: 176.03,74.55 176.24,74.8
S$1587
  Bottom 0: 176.24,74.8 176.36,75.09
S$1588
  Bottom 0: 176.36,75.09 176.41,75.42
S$1589
  Bottom 0: 176.41,75.42 176.36,75.73
S$1590
  Bottom 0: 176.36,75.73 176.24,76.03
S$1591
  Bottom 0: 176.24,76.03 176.03,76.29
S$1592
  Bottom 0: 176.03,76.29 175.76,76.48
S$1593
  Bottom 0: 175.76,76.48 175.46,76.58
S$1594
  Bottom 0: 175.46,76.58 175.37,76.59
S$1595
  Bottom 0: 175.37,76.59 175.37,77.82
S$1596
  Bottom 0: 175.37,77.82 175.58,77.6
S$1597
  Bottom 0: 175.58,77.6 175.87,77.41
S$1598
  Bottom 0: 175.87,77.41 176.2,77.31
S$1599
  Bottom 0: 176.2,77.31 176.55,77.28
S$1600
  Bottom 0: 176.55,77.28 176.9,77.35
S$1601
  Bottom 0: 176.9,77.35 177.21,77.5
S$1602
  Bottom 0: 177.21,77.5 177.48,77.72
S$1603
  Bottom 0: 177.48,77.72 177.69,78.01
S$1604
  Bottom 0: 177.69,78.01 177.78,78.23
S$1605
  Bottom 0: 177.78,78.23 188.23,78.23
S$1606
  Bottom 0: 188.23,78.23 188.3,78.24
S$1607
  Bottom 0: 188.3,78.24 188.37,78.25
S$1608
  Bottom 0: 188.37,78.25 188.43,78.28
S$1609
  Bottom 0: 188.43,78.28 188.49,78.32
S$1610
  Bottom 0: 188.49,78.32 188.55,78.36
S$1611
  Bottom 0: 188.55,78.36 189.41,79.23
S$1612
  Bottom 0: 189.41,79.23 189.51,79.19
S$1613
  Bottom 0: 189.51,79.19 189.82,79.17
S$1614
  Bottom 0: 189.82,79.17 190.11,79.24
S$1615
  Bottom 0: 190.11,79.24 190.38,79.39
S$1616
  Bottom 0: 190.38,79.39 190.58,79.61
S$1617
  Bottom 0: 190.58,79.61 190.71,79.89
S$1618
  Bottom 0: 190.71,79.89 190.76,80.19
S$1619
  Bottom 0: 190.76,80.19 190.71,80.48
S$1620
  Bottom 0: 190.71,80.48 190.58,80.76
S$1621
  Bottom 0: 190.58,80.76 190.38,80.98
S$1622
  Bottom 0: 190.38,80.98 190.11,81.13
S$1623
  Bottom 0: 190.11,81.13 189.82,81.2
S$1624
  Bottom 0: 189.82,81.2 189.51,81.18
S$1625
  Bottom 0: 189.51,81.18 189.23,81.06
S$1626
  Bottom 0: 189.23,81.06 188.99,80.88
S$1627
  Bottom 0: 188.99,80.88 188.83,80.63
S$1628
  Bottom 0: 188.83,80.63 188.74,80.34
S$1629
  Bottom 0: 188.74,80.34 188.74,80.03
S$1630
  Bottom 0: 188.74,80.03 188.79,79.86
S$1631
  Bottom 0: 188.79,79.86 188.04,79.12
S$1632
  Bottom 0: 188.04,79.12 177.78,79.12
S$1633
  Bottom 0: 177.78,79.12 177.69,79.35
S$1634
  Bottom 0: 177.69,79.35 177.48,79.63
S$1635
  Bottom 0: 177.48,79.63 177.21,79.86
S$1636
  Bottom 0: 177.21,79.86 176.9,80.01
S$1637
  Bottom 0: 176.9,80.01 176.55,80.07
S$1638
  Bottom 0: 176.55,80.07 176.2,80.05
S$1639
  Bottom 0: 176.2,80.05 175.87,79.94
S$1640
  Bottom 0: 175.87,79.94 175.58,79.75
S$1641
  Bottom 0: 175.58,79.75 175.37,79.53
S$1642
  Bottom 0: 175.37,79.53 175.37,84.58
S$1643
  Bottom 0: 175.37,84.58 178.05,87.25
S$1644
  Bottom 0: 178.05,87.25 178.08,87.31
S$1645
  Bottom 0: 178.08,87.31 178.12,87.35
S$1646
  Bottom 0: 178.12,87.35 178.13,87.39
S$1647
  Bottom 0: 178.13,87.39 178.16,87.45
S$1648
  Bottom 0: 178.16,87.45 178.16,87.51
S$1649
  Bottom 0: 178.16,87.51 178.18,87.57
S$1650
  Bottom 0: 178.18,87.57 178.18,87.69
S$1651
  Bottom 0: 178.18,87.69 178.62,87.69
S$1652
  Bottom 0: 178.62,87.69 178.7,87.7
S$1653
  Bottom 0: 178.7,87.7 178.77,87.74
S$1654
  Bottom 0: 178.77,87.74 178.83,87.8
S$1655
  Bottom 0: 178.83,87.8 178.87,87.87
S$1656
  Bottom 0: 178.87,87.87 178.88,87.95
S$1657
  Bottom 0: 178.88,87.95 178.88,89.65
S$1658
  Bottom 0: 178.88,89.65 179.49,89.65
S$1659
  Bottom 0: 179.49,89.65 179.32,89.46
S$1660
  Bottom 0: 179.32,89.46 179.18,89.16
S$1661
  Bottom 0: 179.18,89.16 179.13,88.84
S$1662
  Bottom 0: 179.13,88.84 179.18,88.52
S$1663
  Bottom 0: 179.18,88.52 179.32,88.22
S$1664
  Bottom 0: 179.32,88.22 179.53,87.97
S$1665
  Bottom 0: 179.53,87.97 179.8,87.8
S$1666
  Bottom 0: 179.8,87.8 180.11,87.7
S$1667
  Bottom 0: 180.11,87.7 180.44,87.7
S$1668
  Bottom 0: 180.44,87.7 180.75,87.8
S$1669
  Bottom 0: 180.75,87.8 181.02,87.97
S$1670
  Bottom 0: 181.02,87.97 181.24,88.22
S$1671
  Bottom 0: 181.24,88.22 181.37,88.52
S$1672
  Bottom 0: 181.37,88.52 181.42,88.84
S$1673
  Bottom 0: 181.42,88.84 181.37,89.16
S$1674
  Bottom 0: 181.37,89.16 181.24,89.46
S$1675
  Bottom 0: 181.24,89.46 181.06,89.65
S$1676
  Bottom 0: 181.06,89.65 187.26,89.65
S$1677
  Bottom 0: 187.26,89.65 188.79,88.12
S$1678
  Bottom 0: 188.79,88.12 188.74,87.96
S$1679
  Bottom 0: 188.74,87.96 188.74,87.65
S$1680
  Bottom 0: 188.74,87.65 188.83,87.36
S$1681
  Bottom 0: 188.83,87.36 188.99,87.11
S$1682
  Bottom 0: 188.99,87.11 189.23,86.93
S$1683
  Bottom 0: 189.23,86.93 189.51,86.81
S$1684
  Bottom 0: 189.51,86.81 189.82,86.79
S$1685
  Bottom 0: 189.82,86.79 190.11,86.86
S$1686
  Bottom 0: 190.11,86.86 190.38,87.01
S$1687
  Bottom 0: 190.38,87.01 190.58,87.23
S$1688
  Bottom 0: 190.58,87.23 190.71,87.51
S$1689
  Bottom 0: 190.71,87.51 190.76,87.81
S$1690
  Bottom 0: 190.76,87.81 190.71,88.11
S$1691
  Bottom 0: 190.71,88.11 190.58,88.38
S$1692
  Bottom 0: 190.58,88.38 190.38,88.6
S$1693
  Bottom 0: 190.38,88.6 190.11,88.75
S$1694
  Bottom 0: 190.11,88.75 189.82,88.82
S$1695
  Bottom 0: 189.82,88.82 189.51,88.8
S$1696
  Bottom 0: 189.51,88.8 189.41,88.76
S$1697
  Bottom 0: 189.41,88.76 187.76,90.41
S$1698
  Bottom 0: 187.76,90.41 187.71,90.45
S$1699
  Bottom 0: 187.71,90.45 187.65,90.49
S$1700
  Bottom 0: 187.65,90.49 187.59,90.52
S$1701
  Bottom 0: 187.59,90.52 187.52,90.53
S$1702
  Bottom 0: 187.52,90.53 187.45,90.54
S$1703
  Bottom 0: 187.45,90.54 81.04,90.54
S$1704
  Bottom 0: 81.04,90.54 80.97,90.53
S$1705
  Bottom 0: 80.97,90.53 80.9,90.52
S$1706
  Bottom 0: 80.9,90.52 80.84,90.49
S$1707
  Bottom 0: 80.84,90.49 80.78,90.45
S$1708
  Bottom 0: 80.78,90.45 80.72,90.41
S$1709
  Bottom 0: 80.72,90.41 59.19,68.89
S$1710
  Bottom 0: 59.19,68.89 57.14,68.89
S$1711
  Bottom 0: 57.14,68.89 57.2,68.92
S$1712
  Bottom 0: 57.2,68.92 57.41,69.16
S$1713
  Bottom 0: 57.41,69.16 57.55,69.47
S$1714
  Bottom 0: 57.55,69.47 57.59,69.79
S$1715
  Bottom 0: 57.59,69.79 57.55,70.11
S$1716
  Bottom 0: 57.55,70.11 57.41,70.41
S$1717
  Bottom 0: 57.41,70.41 57.2,70.65
S$1718
  Bottom 0: 57.2,70.65 56.92,70.83
S$1719
  Bottom 0: 56.92,70.83 56.61,70.92
S$1720
  Bottom 0: 56.61,70.92 56.29,70.92
S$1721
  Bottom 0: 56.29,70.92 55.98,70.83
S$1722
  Bottom 0: 55.98,70.83 55.7,70.65
S$1723
  Bottom 0: 55.7,70.65 55.49,70.41
S$1724
  Bottom 0: 55.49,70.41 55.35,70.11
S$1725
  Bottom 0: 55.35,70.11 55.31,69.79
S$1726
  Bottom 0: 55.31,69.79 55.35,69.47
S$1727
  Bottom 0: 55.35,69.47 55.49,69.16
S$1728
  Bottom 0: 55.49,69.16 55.7,68.92
S$1729
  Bottom 0: 55.7,68.92 55.76,68.89
S$1730
  Bottom 0: 55.76,68.89 55.05,68.89
S$1731
  Bottom 0: 55.05,68.89 55.05,70.67
S$1732
  Bottom 0: 55.05,70.67 55.04,70.75
S$1733
  Bottom 0: 55.04,70.75 55,70.82
S$1734
  Bottom 0: 55,70.82 54.95,70.88
S$1735
  Bottom 0: 54.95,70.88 54.87,70.92
S$1736
  Bottom 0: 54.87,70.92 54.8,70.93
S$1737
  Bottom 0: 54.8,70.93 54.35,70.93
S$1738
  Bottom 0: 54.35,70.93 54.35,71.06
S$1739
  Bottom 0: 54.35,71.06 54.29,71.28
S$1740
  Bottom 0: 54.29,71.28 54.13,71.44
S$1741
  Bottom 0: 54.13,71.44 53.91,71.5
S$1742
  Bottom 0: 53.91,71.5 53.54,71.5
S$1743
  Bottom 0: 53.54,71.5 52.46,72.59
S$1744
  Bottom 0: 52.46,72.59 52.52,72.73
S$1745
  Bottom 0: 52.52,72.73 52.57,73.05
S$1746
  Bottom 0: 52.57,73.05 52.52,73.37
S$1747
  Bottom 0: 52.52,73.37 52.4,73.67
S$1748
  Bottom 0: 52.4,73.67 52.19,73.92
S$1749
  Bottom 0: 52.19,73.92 51.92,74.11
S$1750
  Bottom 0: 51.92,74.11 51.62,74.22
S$1751
  Bottom 0: 51.62,74.22 51.3,74.24
S$1752
  Bottom 0: 51.3,74.24 50.98,74.17
S$1753
  Bottom 0: 50.98,74.17 50.68,74.02
S$1754
  Bottom 0: 50.68,74.02 50.45,73.8
S$1755
  Bottom 0: 50.45,73.8 50.28,73.53
S$1756
  Bottom 0: 50.28,73.53 50.19,73.21
S$1757
  Bottom 0: 50.19,73.21 50.19,72.89
S$1758
  Bottom 0: 50.19,72.89 50.28,72.57
S$1759
  Bottom 0: 50.28,72.57 50.45,72.3
S$1760
  Bottom 0: 50.45,72.3 50.68,72.07
S$1761
  Bottom 0: 50.68,72.07 50.98,71.92
S$1762
  Bottom 0: 50.98,71.92 51.3,71.86
S$1763
  Bottom 0: 51.3,71.86 51.62,71.88
S$1764
  Bottom 0: 51.62,71.88 51.84,71.96
S$1765
  Bottom 0: 51.84,71.96 52.9,70.89
S$1766
  Bottom 0: 52.9,70.89 52.87,70.88
S$1767
  Bottom 0: 52.87,70.88 52.82,70.82
S$1768
  Bottom 0: 52.82,70.82 52.78,70.75
S$1769
  Bottom 0: 52.78,70.75 52.77,70.67
S$1770
  Bottom 0: 52.77,70.67 52.77,69.24
S$1771
  Bottom 0: 52.77,69.24 51.81,70.2
S$1772
  Bottom 0: 51.81,70.2 51.75,70.24
S$1773
  Bottom 0: 51.75,70.24 51.69,70.28
S$1774
  Bottom 0: 51.69,70.28 51.63,70.31
S$1775
  Bottom 0: 51.63,70.31 51.56,70.32
S$1776
  Bottom 0: 51.56,70.32 51.49,70.33
S$1777
  Bottom 0: 51.49,70.33 39.45,70.33
S$1778
  Bottom 0: 39.45,70.33 39.38,70.32
S$1779
  Bottom 0: 39.38,70.32 39.31,70.31
S$1780
  Bottom 0: 39.31,70.31 39.25,70.28
S$1781
  Bottom 0: 39.25,70.28 39.19,70.24
S$1782
  Bottom 0: 39.19,70.24 39.13,70.2
S$1783
  Bottom 0: 39.13,70.2 38.51,69.58
S$1784
  Bottom 0: 38.51,69.58 38.54,69.79
S$1785
  Bottom 0: 38.54,69.79 38.5,70.11
S$1786
  Bottom 0: 38.5,70.11 38.36,70.41
S$1787
  Bottom 0: 38.36,70.41 38.15,70.65
S$1788
  Bottom 0: 38.15,70.65 37.87,70.83
S$1789
  Bottom 0: 37.87,70.83 37.56,70.92
S$1790
  Bottom 0: 37.56,70.92 37.24,70.92
S$1791
  Bottom 0: 37.24,70.92 36.93,70.83
S$1792
  Bottom 0: 36.93,70.83 36.65,70.65
S$1793
  Bottom 0: 36.65,70.65 36.44,70.41
S$1794
  Bottom 0: 36.44,70.41 36.3,70.11
S$1795
  Bottom 0: 36.3,70.11 36.26,69.79
S$1796
  Bottom 0: 36.26,69.79 36.3,69.47
S$1797
  Bottom 0: 36.3,69.47 36.44,69.16
S$1798
  Bottom 0: 36.44,69.16 36.65,68.92
S$1799
  Bottom 0: 36.65,68.92 36.76,68.86
S$1800
  Bottom 0: 36.76,68.86 36,68.86
S$1801
  Bottom 0: 36,68.86 36.01,68.9
S$1802
  Bottom 0: 36.01,68.9 36.01,70.67
S$1803
  Bottom 0: 36.01,70.67 35.99,70.75
S$1804
  Bottom 0: 35.99,70.75 35.95,70.82
S$1805
  Bottom 0: 35.95,70.82 35.9,70.88
S$1806
  Bottom 0: 35.9,70.88 35.83,70.92
S$1807
  Bottom 0: 35.83,70.92 35.75,70.93
S$1808
  Bottom 0: 35.75,70.93 35.3,70.93
S$1809
  Bottom 0: 35.3,70.93 35.3,71.06
S$1810
  Bottom 0: 35.3,71.06 35.24,71.28
S$1811
  Bottom 0: 35.24,71.28 35.08,71.44
S$1812
  Bottom 0: 35.08,71.44 34.86,71.5
S$1813
  Bottom 0: 34.86,71.5 34.5,71.5
S$1814
  Bottom 0: 34.5,71.5 33.41,72.59
S$1815
  Bottom 0: 33.41,72.59 33.48,72.72
S$1816
  Bottom 0: 33.48,72.72 33.52,73.04
S$1817
  Bottom 0: 33.52,73.04 33.48,73.36
S$1818
  Bottom 0: 33.48,73.36 33.35,73.66
S$1819
  Bottom 0: 33.35,73.66 33.14,73.92
S$1820
  Bottom 0: 33.14,73.92 32.88,74.11
S$1821
  Bottom 0: 32.88,74.11 32.57,74.21
S$1822
  Bottom 0: 32.57,74.21 32.24,74.23
S$1823
  Bottom 0: 32.24,74.23 31.93,74.17
S$1824
  Bottom 0: 31.93,74.17 31.64,74.02
S$1825
  Bottom 0: 31.64,74.02 31.4,73.8
S$1826
  Bottom 0: 31.4,73.8 31.23,73.52
S$1827
  Bottom 0: 31.23,73.52 31.14,73.2
S$1828
  Bottom 0: 31.14,73.2 31.14,72.88
S$1829
  Bottom 0: 31.14,72.88 31.23,72.56
S$1830
  Bottom 0: 31.23,72.56 31.4,72.29
S$1831
  Bottom 0: 31.4,72.29 31.64,72.07
S$1832
  Bottom 0: 31.64,72.07 31.93,71.92
S$1833
  Bottom 0: 31.93,71.92 32.24,71.85
S$1834
  Bottom 0: 32.24,71.85 32.57,71.87
S$1835
  Bottom 0: 32.57,71.87 32.79,71.95
S$1836
  Bottom 0: 32.79,71.95 33.85,70.89
S$1837
  Bottom 0: 33.85,70.89 33.83,70.88
S$1838
  Bottom 0: 33.83,70.88 33.77,70.82
S$1839
  Bottom 0: 33.77,70.82 33.73,70.75
S$1840
  Bottom 0: 33.73,70.75 33.72,70.67
S$1841
  Bottom 0: 33.72,70.67 33.72,68.9
S$1842
  Bottom 0: 33.72,68.9 33.72,68.86
S$1843
  Bottom 0: 33.72,68.86 27.61,68.86
S$1844
  Bottom 0: 27.61,68.86 27.58,69.06
S$1845
  Bottom 0: 27.58,69.06 27.45,69.33
S$1846
  Bottom 0: 27.45,69.33 27.24,69.55
S$1847
  Bottom 0: 27.24,69.55 26.98,69.7
S$1848
  Bottom 0: 26.98,69.7 26.68,69.76
S$1849
  Bottom 0: 26.68,69.76 26.38,69.75
S$1850
  Bottom 0: 26.38,69.75 26.1,69.63
S$1851
  Bottom 0: 26.1,69.63 25.86,69.45
S$1852
  Bottom 0: 25.86,69.45 25.69,69.2
S$1853
  Bottom 0: 25.69,69.2 25.6,68.91
S$1854
  Bottom 0: 25.6,68.91 25.6,68.64
S$1855
  Bottom 0: 25.6,68.64 25.58,68.66
S$1856
  Bottom 0: 25.58,68.66 25.58,75.24
S$1857
  Bottom 0: 25.58,75.24 25.57,75.31
S$1858
  Bottom 0: 25.57,75.31 25.56,75.37
S$1859
  Bottom 0: 25.56,75.37 25.53,75.44
S$1860
  Bottom 0: 25.53,75.44 25.49,75.5
S$1861
  Bottom 0: 25.49,75.5 25.45,75.55
S$1862
  Bottom 0: 25.45,75.55 23.65,77.36
S$1863
  Bottom 0: 23.65,77.36 23.8,77.31
S$1864
  Bottom 0: 23.8,77.31 24.15,77.28
S$1865
  Bottom 0: 24.15,77.28 24.5,77.35
S$1866
  Bottom 0: 24.5,77.35 24.81,77.5
S$1867
  Bottom 0: 24.81,77.5 25.08,77.72
S$1868
  Bottom 0: 25.08,77.72 25.29,78.01
S$1869
  Bottom 0: 25.29,78.01 25.38,78.23
S$1870
  Bottom 0: 25.38,78.23 31.48,78.23
S$1871
  Bottom 0: 31.48,78.23 31.55,78.24
S$1872
  Bottom 0: 31.55,78.24 31.62,78.25
S$1873
  Bottom 0: 31.62,78.25 31.68,78.28
S$1874
  Bottom 0: 31.68,78.28 31.74,78.32
S$1875
  Bottom 0: 31.74,78.32 31.8,78.36
S$1876
  Bottom 0: 31.8,78.36 34.02,80.58
S$1877
  Bottom 0: 34.02,80.58 33.94,80.34
S$1878
  Bottom 0: 33.94,80.34 33.94,80.03
S$1879
  Bottom 0: 33.94,80.03 34.03,79.74
S$1880
  Bottom 0: 34.03,79.74 34.2,79.49
S$1881
  Bottom 0: 34.2,79.49 34.44,79.31
S$1882
  Bottom 0: 34.44,79.31 34.72,79.19
S$1883
  Bottom 0: 34.72,79.19 35.02,79.17
S$1884
  Bottom 0: 35.02,79.17 35.32,79.24
S$1885
  Bottom 0: 35.32,79.24 35.58,79.39
S$1886
  Bottom 0: 35.58,79.39 35.78,79.61
S$1887
  Bottom 0: 35.78,79.61 35.92,79.89
S$1888
  Bottom 0: 35.92,79.89 35.96,80.19
S$1889
  Bottom 0: 35.96,80.19 35.92,80.48
S$1890
  Bottom 0: 35.92,80.48 35.78,80.76
S$1891
  Bottom 0: 35.78,80.76 35.66,80.89
S$1892
  Bottom 0: 35.66,80.89 35.99,80.89
S$1893
  Bottom 0: 35.99,80.89 36.38,80.51
S$1894
  Bottom 0: 36.38,80.51 36.32,80.34
S$1895
  Bottom 0: 36.32,80.34 36.32,80.03
S$1896
  Bottom 0: 36.32,80.03 36.41,79.74
S$1897
  Bottom 0: 36.41,79.74 36.58,79.49
S$1898
  Bottom 0: 36.58,79.49 36.82,79.31
S$1899
  Bottom 0: 36.82,79.31 37.09,79.19
S$1900
  Bottom 0: 37.09,79.19 37.4,79.17
S$1901
  Bottom 0: 37.4,79.17 37.69,79.24
S$1902
  Bottom 0: 37.69,79.24 37.96,79.39
S$1903
  Bottom 0: 37.96,79.39 38.16,79.61
S$1904
  Bottom 0: 38.16,79.61 38.29,79.89
S$1905
  Bottom 0: 38.29,79.89 38.34,80.19
S$1906
  Bottom 0: 38.34,80.19 38.29,80.48
S$1907
  Bottom 0: 38.29,80.48 38.16,80.76
S$1908
  Bottom 0: 38.16,80.76 37.96,80.98
S$1909
  Bottom 0: 37.96,80.98 37.69,81.13
S$1910
  Bottom 0: 37.69,81.13 37.4,81.2
S$1911
  Bottom 0: 37.4,81.2 37.09,81.18
S$1912
  Bottom 0: 37.09,81.18 36.99,81.14
S$1913
  Bottom 0: 36.99,81.14 36.48,81.65
S$1914
  Bottom 0: 36.48,81.65 36.43,81.69
S$1915
  Bottom 0: 36.43,81.69 36.37,81.73
S$1916
  Bottom 0: 36.37,81.73 36.31,81.75
S$1917
  Bottom 0: 36.31,81.75 36.24,81.77
S$1918
  Bottom 0: 36.24,81.77 36.17,81.78
S$1919
  Bottom 0: 36.17,81.78 34.14,81.78
S$1920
